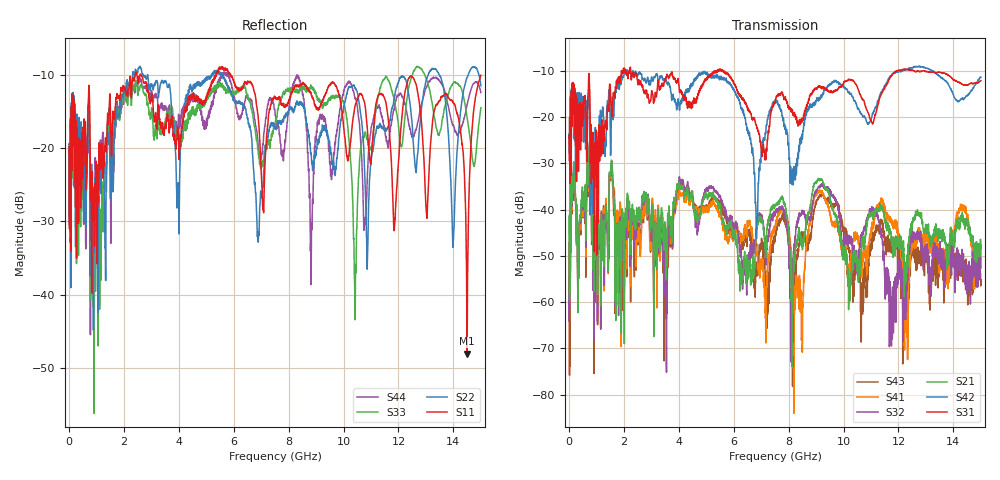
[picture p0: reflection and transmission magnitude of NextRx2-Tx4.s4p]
! FILE: N:\QM 2007\Prüfprotokolle\Highspeed\Konfektionierte Ltg\L45593-D106\D30\8216\0002\Next  Platine 2\NextRx2-Tx4.s4p
# MHz S DB R 50.00
! FREQ  S11  S12  S13  S14
!  S21  S22  S23  S24
!  S31  S32  S33  S34
!  S41  S42  S43  S44
!  DB  ANG  DB  ANG  DB  ANG  DB  ANG
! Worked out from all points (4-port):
!   2999 points, 10 MHz to 15 GHz, reference 50 ohm
!   strongest paths, dB at 10 MHz, 3.755 GHz, 7.505 GHz, 11.26 GHz, 15 GHz:
!     S31: -24.1, -10.2, -16.6, -17.1, -12.1
!     S42: -23.7, -15.9, -17.1, -16.7, -11.4
!     S21: -41.6, -42.3, -39.2, -40.5, -48.4
!     S32: -59.2, -43.0, -40.9, -41.2, -50.4
!     S41: -57.3, -42.7, -43.9, -39.4, -47.7
!     S43: -47.3, -44.2, -47.0, -44.4, -55.2
!   lowest |S11| = -48.1 dB at 14.49 GHz (marker M1), VSWR 1.01, Z = 50.1 - j0.388 ohm
!   |S11| at or under -10 dB: start of sweep to 2.416 GHz; 2.635 GHz to 5.361 GHz (2.725 GHz wide, 68.2 % of centre); 5.89 GHz to end of sweep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
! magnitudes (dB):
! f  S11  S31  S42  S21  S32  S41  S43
! 10 MHz  -19.8  -24.1  -23.7  -41.6  -59.2  -57.3  -47.3
! 735 MHz  -11.4  -10.9  -15.0  -29.2  -29.6  -29.1  -29.9
! 8.47 GHz  -11.3  -20.3  -25.2  -47.3  -40.9  -68.3  -45.4
! 9.105 GHz  -14.4  -13.4  -15.8  -33.6  -35.2  -36.0  -37.1
! 12.28 GHz  -11.5  -9.7  -9.8  -52.8  -56.3  -64.8  -54.7
! 14.49 GHz  -48.1  -13.1  -15.4  -43.6  -52.0  -41.4  -58.1
! 15 GHz  -10.0  -12.1  -11.4  -48.4  -50.4  -47.7  -55.2
